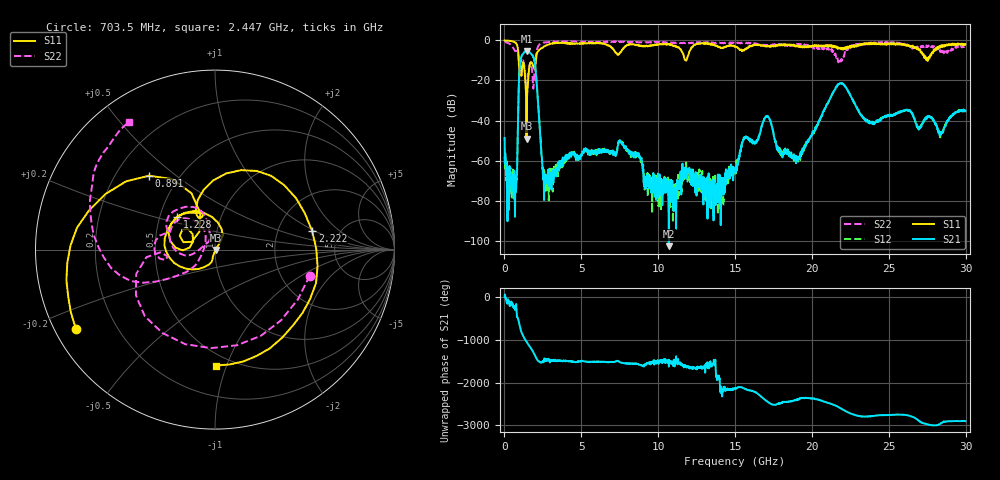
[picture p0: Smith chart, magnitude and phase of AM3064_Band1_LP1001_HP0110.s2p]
# Hz S DB R 50.0
!freq dBS11 angS11 dBS21 angS21 dBS12 angS12 dBS22 angS22
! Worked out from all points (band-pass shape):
!   1600 points, 10 MHz to 29.98 GHz, reference 50 ohm
!   highest |S21| = -5.21 dB at 1.453 GHz (marker M1); lowest = -102.8 dB at 10.69 GHz (marker M2)
!   |S21| within 3 dB of the highest: 1.097 GHz to 1.873 GHz (776 MHz wide, 52.3 % of centre)
!   lowest |S11| = -49.1 dB at 1.435 GHz (marker M3), VSWR 1.01, Z = 50.3 - j0.166 ohm
!   |S11| at or under -10 dB: 931.5 MHz to 2.044 GHz (1.112 GHz wide, 74.8 % of centre); 11.78906 GHz to 11.83726 GHz (48.19 MHz wide, 0.408 % of centre); 27.52132 GHz to 27.54925 GHz (27.93 MHz wide, 0.101 % of centre)
!   |S22| runs from -25.0 to -0.4 dB; largest |S21 - S12| = 0.0058
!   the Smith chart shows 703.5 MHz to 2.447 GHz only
!   S11 on the Smith chart (normalised r, x): 703.5 MHz: 0.06, -0.26; 891 MHz: 0.34, +0.40; 1.228 GHz: 0.62, +0.24; 2.222 GHz: 3.16, +0.93; 2.447 GHz: 0.41, -0.92
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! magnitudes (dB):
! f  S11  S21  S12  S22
! 10 MHz  0.0  -48.7  -57.9  -0.4
! 703.5 MHz  -1.0  -71.6  -68.4  -5.2
! 891 MHz  -5.2  -35.3  -35.4  -6.8
! 1.041 GHz  -13.4  -10.3  -10.2  -9.5
! 1.228 GHz  -11.1  -6.5  -6.5  -10.4
! 1.435 GHz  -49.1  -5.2  -5.2  -25.0
! 1.453 GHz  -32.8  -5.2  -5.2  -24.6
! 1.922 GHz  -13.6  -9.3  -9.3  -19.0
! 2.222 GHz  -5.2  -35.1  -35.0  -2.5
! 2.447 GHz  -3.8  -60.2  -59.5  -1.3
! 2.784 GHz  -2.3  -67.8  -68.2  -0.9
! 5.015 GHz  -1.4  -57.5  -57.0  -0.8
! 7.564 GHz  -5.9  -50.7  -50.7  -0.5
! 10 GHz  -2.0  -77.4  -69.9  -0.9
! 10.69 GHz  -1.9  -102.8  -70.9  -1.1
! 15 GHz  -3.0  -63.7  -64.6  -1.4
! 17.05 GHz  -2.8  -37.9  -37.8  -2.5
! 18.98 GHz  -2.5  -57.9  -59.3  -2.2
! 19.99 GHz  -3.1  -47.0  -46.7  -3.0
! 21.85 GHz  -3.7  -21.4  -21.3  -11.1
! 25 GHz  -1.4  -37.6  -37.6  -1.1
! 29.98 GHz  -1.9  -35.2  -35.2  -3.1
